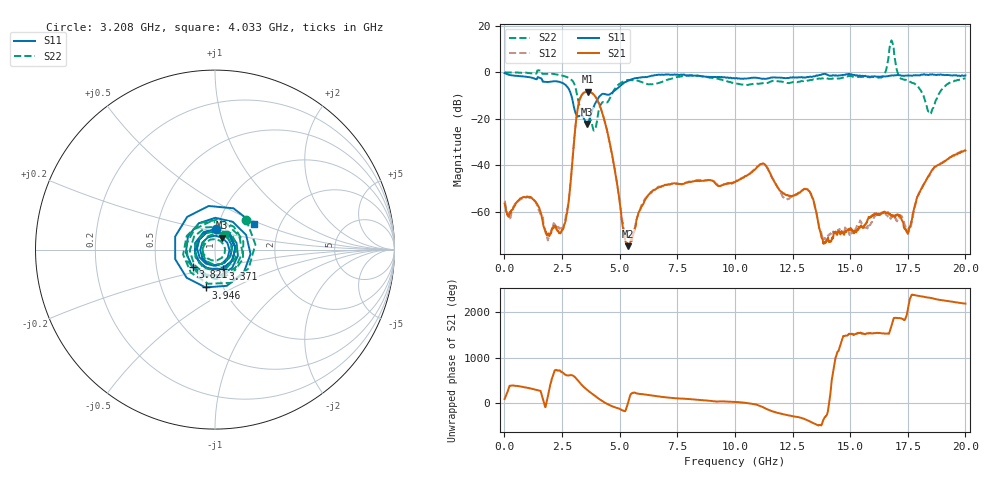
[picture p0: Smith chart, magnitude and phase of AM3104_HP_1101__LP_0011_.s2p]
!Created with skrf (http://scikit-rf.org).
# Hz S RI R 50.0
!freq ReS11 ImS11 ReS21 ImS21 ReS12 ImS12 ReS22 ImS22
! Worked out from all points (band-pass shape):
!   1601 points, 10 MHz to 20 GHz, reference 50 ohm
!   highest |S21| = -8.28 dB at 3.608 GHz (marker M1); lowest = -74.7 dB at 5.357 GHz (marker M2)
!   |S21| within 3 dB of the highest: 3.284 GHz to 3.999 GHz (715.6 MHz wide, 19.6 % of centre)
!   lowest |S11| = -22.2 dB at 3.596 GHz (marker M3), VSWR 1.17, Z = 53.6 + j7.18 ohm
!   |S11| at or under -10 dB: 2.907 GHz to 4.158 GHz (1.251 GHz wide, 35.4 % of centre)
!   |S22| runs from -25.0 to 13.7 dB; largest |S21 - S12| = 0.014
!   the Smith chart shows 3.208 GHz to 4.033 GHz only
!   S11 on the Smith chart (normalised r, x): 3.208 GHz: 0.99, +0.23; 3.371 GHz: 1.07, -0.23; 3.821 GHz: 0.77, -0.15; 3.946 GHz: 0.83, -0.37; 4.033 GHz: 1.47, +0.45
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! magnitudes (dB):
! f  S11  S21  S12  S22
! 10 MHz  -0.4  -56.3  -55.2  0.0
! 1.109 GHz  -2.2  -53.5  -53.9  -0.4
! 2.471 GHz  -4.4  -68.2  -67.9  -1.3
! 2.746 GHz  -6.5  -58.6  -57.8  -2.2
! 3.208 GHz  -18.9  -14.2  -14.2  -12.4
! 3.346 GHz  -18.9  -9.9  -10.0  -15.7
! 3.371 GHz  -18.7  -9.6  -9.6  -15.7
! 3.596 GHz  -22.2  -8.3  -8.4  -17.9
! 3.608 GHz  -22.1  -8.3  -8.4  -18.1
! 3.821 GHz  -16.0  -9.1  -9.1  -23.2
! 3.946 GHz  -13.3  -10.4  -10.5  -24.1
! 4.033 GHz  -11.8  -11.9  -11.9  -19.9
! 5.357 GHz  -3.7  -74.7  -70.5  -3.3
! 6.682 GHz  -1.1  -49.6  -49.1  -4.7
! 10.01 GHz  -2.7  -47.2  -47.1  -4.8
! 11.2 GHz  -2.8  -39.2  -39.3  -4.7
! 13.34 GHz  -2.0  -53.4  -53.4  -3.3
! 13.9 GHz  -0.7  -73.0  -71.2  -2.4
! 16.68 GHz  -1.5  -60.7  -62.2  7.2
! 17.53 GHz  -1.4  -68.7  -68.2  -3.6
! 18.45 GHz  -1.0  -43.6  -44.2  -17.3
! 20 GHz  -1.4  -33.6  -33.0  -2.7
